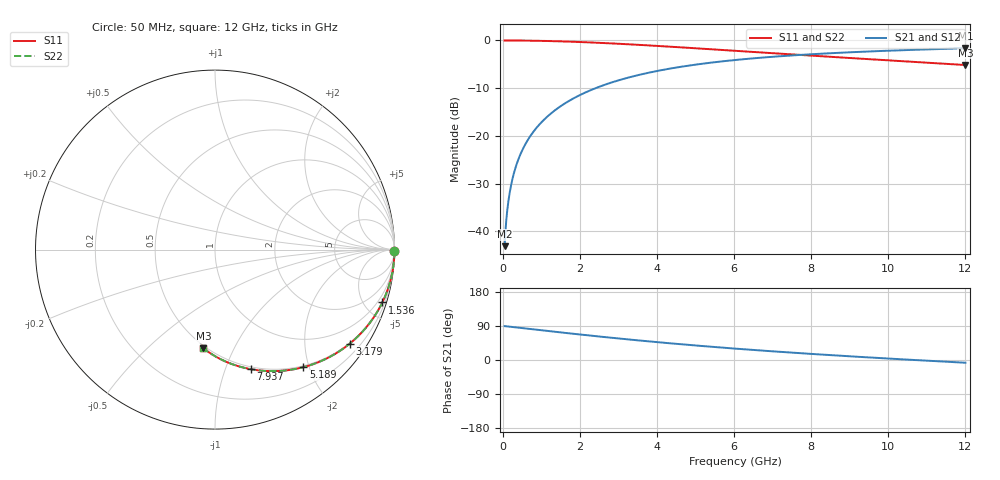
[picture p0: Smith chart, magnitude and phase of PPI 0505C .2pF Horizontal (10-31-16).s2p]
# MHz S MA R 50
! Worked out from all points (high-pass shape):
!   1601 points, 50 MHz to 12 GHz, reference 50 ohm
!   highest |S21| = -1.64 dB at 12 GHz (marker M1); lowest = -43.1 dB at 50 MHz (marker M2)
!   |S21| within 3 dB of the highest: 5.412 GHz to end of sweep
!   lowest |S11| = -5.1 dB at 12 GHz (marker M3), VSWR 3.47, Z = 24.2 - j38.2 ohm
!   |S11| at or under -10 dB: nowhere
!   |S22| runs from -5.1 to 0.0 dB; largest |S21 - S12| = 0
!   S11 on the Smith chart (normalised r, x): 50 MHz: open; 1.536 GHz: 0.48, -6.45; 3.179 GHz: 0.48, -3.12; 5.189 GHz: 0.48, -1.91; 7.937 GHz: 0.48, -1.23; 12 GHz: 0.48, -0.76
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50  1 -0.6  0.006981 89.4  0.006981 89.4  1 -0.6
79.875  0.9999 -0.9  0.01115 89.1  0.01115 89.1  0.9999 -0.9
147.0938  0.9998 -1.7  0.02053 88.3  0.02053 88.3  0.9998 -1.7
176.9688  0.9997 -2.0  0.0247 88.0  0.0247 88.0  0.9997 -2.0
214.3125  0.9995 -2.5  0.02991 87.5  0.02991 87.5  0.9995 -2.5
266.5938  0.9993 -3.1  0.03719 86.9  0.03719 86.9  0.9993 -3.1
326.3438  0.9989 -3.8  0.04551 86.2  0.04551 86.2  0.9989 -3.8
468.25  0.9978 -5.4  0.06522 84.6  0.06522 84.6  0.9978 -5.4
662.4375  0.9957 -7.6  0.09203 82.4  0.09203 82.4  0.9957 -7.6
901.4375  0.9921 -10.4  0.1247 79.6  0.1247 79.6  0.9921 -10.4
1192.719  0.9863 -13.7  0.1639 76.3  0.1639 76.3  0.9863 -13.7
1536.281  0.9777 -17.5  0.2089 72.5  0.2089 72.5  0.9777 -17.5
2044.156  0.9618 -23.1  0.2727 66.9  0.2727 66.9  0.9618 -23.1
2574.438  0.9417 -28.7  0.335 61.2  0.335 61.2  0.9417 -28.7
3179.406  0.9157 -34.9  0.4002 55.1  0.4002 55.1  0.9157 -34.9
4038.312  0.8753 -43.1  0.4816 46.8  0.4816 46.8  0.8753 -43.1
5188.5  0.8192 -53.1  0.571 36.8  0.571 36.8  0.8192 -53.1
6025  0.7794 -59.8  0.6237 30.1  0.6237 30.1  0.7794 -59.8
7937  0.6961 -73.2  0.7143 16.5  0.7143 16.5  0.6961 -73.2
8019.156  0.6928 -73.8  0.7175 16.0  0.7175 16.0  0.6928 -73.8
10013.31  0.6186 -85.9  0.7812 3.8  0.7812 3.8  0.6186 -85.9
12000  0.5528 -96.7  0.8278 -7.2  0.8278 -7.2  0.5528 -96.7
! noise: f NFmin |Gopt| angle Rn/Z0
50  0.004112  0.993  0.5723  0.1356
1372  0.006667  0.844  10.84  0.008991
2701  0.009299  0.7594  16.61  0.00767
4031  0.01178  0.709  21.28  0.007702
5360  0.01416  0.6762  25.62  0.00804
6682  0.01647  0.654  29.78  0.008494
8012  0.01879  0.6387  33.85  0.009018
9341  0.02112  0.6285  37.82  0.009597
1.067e+04  0.0235  0.6224  41.67  0.01023
1.2e+04  0.02595  0.6196  45.41  0.01093
